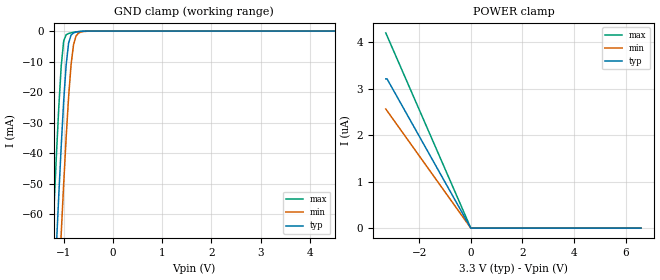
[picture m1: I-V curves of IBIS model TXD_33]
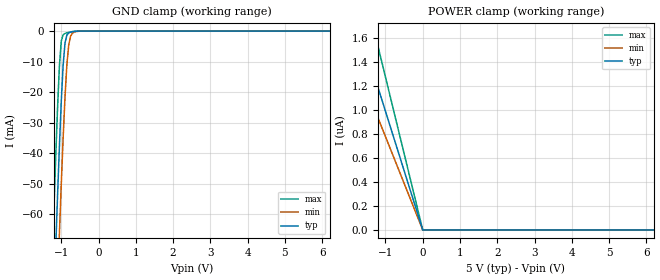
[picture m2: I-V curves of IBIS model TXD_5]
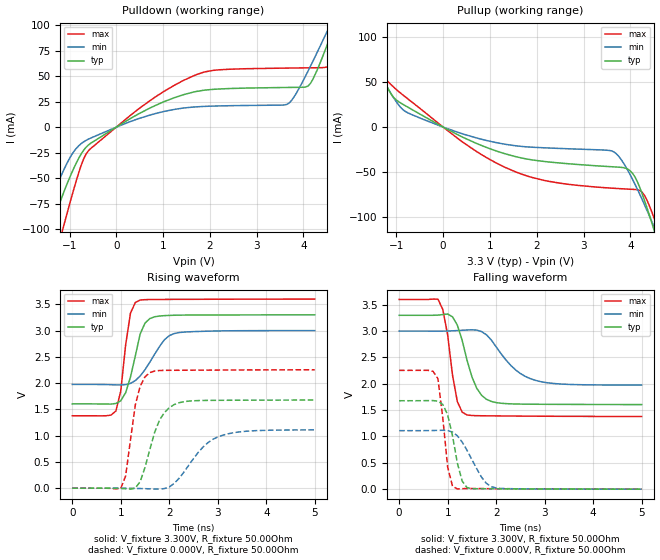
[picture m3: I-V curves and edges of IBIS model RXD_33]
| Texas Instruments Incorporated
| 3000-VRMS Small-Footprint and Low-Power Triple and Quad Channels Digital
| Isolators
| Marketing part#   Digital Voltage Range   Package-type   #pins
| ISO7131CCDBQ   3V - 5.5V   QSOP   16
| ISO7131CCDBQR   3V - 5.5V   QSOP   16
[IBIS Ver]   4.1
[File name]   iso7131.ibs
[File Rev]   1.0
[Date]   04/12/2013
[Source]
| Texas Instruments Incorporated.
| Analog-eLab, HPA
| 12500 TI Blvd
| Dallas, TX -75243
[Notes]   Revision History
| Rev 1.0: 04/12/2013
| - Initial model not matched to silicon
| - C_comp although listed in numberical order of value are
|   obtained from varying PVT conditions.For PVT conditions for
|   eachspecific value, refer to the buffer description under
|   repective [Model].IBIS model user is responsible for using
|   appropriate C_comp to simulate for Signal Integrity.
| - Model names with a trailing _33 contains the model for 3.3V
|   [3.0V and 3.6V]. Model names with a trailing _5 contains the
|   model for 5.0V [4.5V and 5.5V].
[Disclaimer]
| This model is designed as an aid for customers of Texas Instruments.
| TI and its licensors and suppliers make no warranties, either expressed
| or implied, with respect to this  model, including the warranties of
| merchantability or fitness for a particular purpose.
| The model is provided solely on an "as is" basis. The entire risk as to
| its quality and performance is with the customer.
[Copyright] (C)Copyright 2013 Texas Instruments Incorporated.
   All rights reserved.
|   Component ISO7131
[Component]   ISO7131CC
[Manufacturer]  TI
[Package]   |16-pin QSOP  -  DBQ package
|   typ   min   max
R_pkg   0.094432   0.09129   0.09717
L_pkg   1.69628nH   1.65883nH   1.72962nH
C_pkg   0.24832pF   0.2469pF   0.25012pF
[Pin]  signal_name   model_name   R_pin   L_pin   C_pin
1   VCC1   POWER   0.09287  1.67713n  0.24790p
2   GND1   GND   0.05804  1.59222n  0.24871p
3   INA   TXD   0.09129  1.65883n  0.24690p
4   INB   TXD   0.09717  1.72962n  0.24976p
5   OUTC   RXD   0.09664  1.72132n  0.25012p
6   NC   NC   0.03819  1.41587n  0.54383p
7   EN1   NC   0.03819  1.41587n  0.54383p
8   GND1   GND   0.05911  1.64321n  0.24516p
9   GND2   GND   0.05906  1.58357n  0.49660p
10   EN2   NC   0.02805  1.16989n  0.35967p
11   NC   NC   0.02805  1.16989n  0.35967p
12   INC   TXD   0.09546  1.70981n  0.24826p
13   OUTB   RXD   0.09359  1.68659n  0.24766p
14   OUTA   RXD   0.09244  1.67155n  0.24725p
15   GND2   GND   0.03870  1.24255n  0.31586p
16   VCC2   POWER   0.05301  1.30868n  0.31101p
[Model Selector] TXD
TXD_33   TXD Input model for 3.0V - 3.6V
TXD_5   TXD Input model for 4.5V - 5.5V
[Model Selector] RXD
RXD_33   RXD Output model for 3.0V - 3.6V
RXD_5   RXD Output model for 4.5V - 5.5V
| Models and submodels in the file (4): TXD_33 (Input), TXD_5 (Input), RXD_33 (Output), RXD_5 (Output)
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|   TXD_33 Model
[Model]   TXD_33
Model_type   Input
|Signals   TXD
Vinh = 2.0
Vinl = 0.8
|   typ   min   max
|   (nom PVT)   (slow PVT)   (fast PVT)
C_comp   0.6217pF   0.5756pF   0.6712pF
|   typ   min   max
[Voltage Range]   3.3V   3.0V   3.6V
[Temperature Range]   27.0   136.0   -40.0
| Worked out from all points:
|   GND clamp passes 1 mA (typ) near -0.83 V on its own axis
[GND Clamp]
|   Voltage   I(typ)   I(min)   I(max)
-3.3V     -896mA     -941.7mA   -892.3mA
-1.25V    -107.4mA   -137.4mA   -77.4mA
-1.2V     -89.12mA   -119.2mA   -59.18mA
-1.15V    -71.29mA   -101.2mA   -41.62mA
-1.1V     -54.06mA   -83.57mA   -25.26mA
-1.05V    -37.76mA   -66.5mA    -11.46mA
-1V       -23.03mA   -50.19mA   -3.269mA
-950mV    -11.14mA   -35mA      -1.197mA
-900mV    -3.932mA   -21.61mA   -785uA
-800mV    -612.2uA   -4.508mA   -387.7uA
-600mV    -46.68uA   -168.3uA   -47.31uA
6.6V      0A         0A         0A
[POWER Clamp]
|   Voltage   I(typ)   I(min)   I(max)
-3.3V     3.211uA    2.564uA    4.201uA
-3.25V    3.211uA    2.525uA    4.138uA
0V        0A         0A         0A
6.6V      0A         0A         0A
|   TXD_5 Model
[Model]   TXD_5
Model_type   Input
|Signals   TXD
Vinh = 2.0
Vinl = 0.8
|   typ   min   max
|   (nom PVT)   (slow PVT)   (fast PVT)
C_comp   0.5878pF   0.5481pF   0.6309pF
|   typ   min   max
[Voltage Range]   5.0V   4.5V   5.5V
[Temperature Range]   27.0   136.0   -40.0
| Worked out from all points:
|   GND clamp passes 1 mA (typ) near -0.83 V on its own axis
[GND Clamp]
|   Voltage   I(typ)   I(min)   I(max)
-5V       -1.6A      -1.623A    -1.559A
-1.25V    -107.4mA   -137.4mA   -77.4mA
-1.2V     -89.12mA   -119.2mA   -59.18mA
-1.15V    -71.29mA   -101.2mA   -41.62mA
-1.1V     -54.06mA   -83.57mA   -25.26mA
-1.05V    -37.76mA   -66.5mA    -11.46mA
-1V       -23.04mA   -50.19mA   -3.27mA
-950mV    -11.15mA   -35mA      -1.198mA
-850mV    -1.31mA    -11.07mA   -557.5uA
-750mV    -352.2uA   -1.64mA    -261.2uA
-550mV    -20.4uA    -82.68uA   -21.52uA
10V       0A         0A         0A
[POWER Clamp]
|   Voltage   I(typ)   I(min)   I(max)
-5V       4.941uA    3.885uA    6.302uA
-2.15V    2.125uA    1.671uA    2.737uA
-2.1V     2.075uA    1.632uA    2.674uA
-1.7V     1.68uA     1.321uA    2.164uA
-1.65V    1.63uA     1.282uA    2.101uA
-1.3V     1.285uA    1.01uA     1.655uA
0V        0A         0A         0A
10V       0A         0A         0A
|   RXD_33 MODEL
[Model]   RXD_33
Model_type   Output
| Signals   RXD
Vmeas = 1.55V   |Reference voltage for timing measurements
Cref = 15pF   |Timing specification test load capacitance value
| variable   typ   min   max
|   (nom PVT)   (slow PVT)   (fast PVT)
|C_comp Average
C_comp   2.5852pF   2.2483pF   3.0761pF
|C_comp Output Low
|C_comp   2.6504pF   2.3554pF   3.1260pF
|C_comp Output High
|C_comp   2.5200pF   2.1412pF   3.0261pF
|   typ   min   max
[Voltage Range]   3.3V   3.0V   3.6V
[Temperature Range]   27.0   136.0   -40.0
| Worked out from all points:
|   slope of the pulldown table from 0 to 0.495 V, typ, clamps not added: 36.9 ohm
|   slope of the pullup table from 0 to 0.495 V, typ, clamps not added: 38.1 ohm
|   falling waveform, V_fixture 3.300V, R_fixture 50.00Ohm: 20-80 % time 334ps typ, 600ps min, 215ps max; typ from 3.3 V to 1.6 V
|   rising waveform, V_fixture 3.300V, R_fixture 50.00Ohm: 20-80 % time 269ps typ, 440ps min, 178ps max; typ from 1.6 V to 3.3 V
|   rising waveform, V_fixture 0.000V, R_fixture 50.00Ohm: 20-80 % time 354ps typ, 601ps min, 230ps max; typ from 0 V to 1.68 V
|   falling waveform, V_fixture 0.000V, R_fixture 50.00Ohm: 20-80 % time 229ps typ, 400ps min, 158ps max; typ from 1.68 V to 0 V
[Pulldown]
|   Voltage   I(typ)   I(min)   I(max)
-3.3V     -444mA     -323.4mA   -559.5mA
-1.65V    -147.4mA   -102.5mA   -196.8mA
-1.35V    -95.7mA    -66.33mA   -136mA
-1.15V    -67.06mA   -44.62mA   -101.2mA
-600mV    -17.67mA   -11.86mA   -23.39mA
1.65V     34.39mA    19.71mA    50.29mA
3.65V     38.89mA    22.42mA    57.89mA
4.15V     42.92mA    59.74mA    58.14mA
4.55V     85.96mA    98.03mA    60.72mA
4.65V     98.18mA    107.5mA    71.46mA
4.85V     122.5mA    126mA      101.8mA
6.6V      280.4mA    243.7mA    322.1mA
[Pullup]
|   Voltage   I(typ)   I(min)   I(max)
-3.3V     239.5mA    206.9mA    282.1mA
-1.95V    129.9mA    113.6mA    151.3mA
-1.7V     102.1mA    91.19mA    115.7mA
-1.3V     55.75mA    53.78mA    58.94mA
-1V       29.98mA    27.94mA    41.63mA
0V        124.8pA    622.4pA    79.46pA
1.35V     -29.93mA   -19.18mA   -45.19mA
3.65V     -44.04mA   -27.51mA   -67.78mA
4.05V     -51.38mA   -58.2mA    -68.97mA
4.3V      -80.92mA   -85.71mA   -75.5mA
4.55V     -121.4mA   -116mA     -107.4mA
6.6V      -493.8mA   -392mA     -570.7mA
[Ramp]
R_load = 50.00Ohm
|   typ   min   max
dV/dt_r   1.007V/353.701ps 666.318mV/600.696ps   1.353V/229.593ps
dV/dt_f   1.017V/334.234ps 614.806mV/599.733ps   1.333V/215.151ps
[Falling Waveform]
V_fixture = 3.300V
V_fixture_min = 3.000V
V_fixture_max = 3.600V
R_fixture = 50.00Ohm
|   Time   V(typ)   V(min)   V(max)
0s        3.3V       3V         3.6V
800ps     3.304V     3V         3.606V
900ps     3.313V     3V         3.41V
1ns       3.324V     3.001V     2.928V
1.2ns     3.113V     3.01V      1.661V
1.4ns     2.445V     3.021V     1.408V
1.6ns     1.915V     3.019V     1.395V
1.9ns     1.665V     2.831V     1.391V
2.8ns     1.612V     2.068V     1.385V
5ns       1.605V     1.975V     1.379V
[Rising Waveform]
V_fixture = 3.300V
V_fixture_min = 3.000V
V_fixture_max = 3.600V
R_fixture = 50.00Ohm
|   Time   V(typ)   V(min)   V(max)
0s        1.605V     1.975V     1.379V
900ps     1.613V     1.967V     1.471V
1ns       1.664V     1.965V     1.851V
1.1ns     1.817V     1.971V     2.723V
1.2ns     2.114V     1.995V     3.333V
1.4ns     2.937V     2.136V     3.582V
1.6ns     3.229V     2.4V       3.591V
1.9ns     3.284V     2.825V     3.593V
2.1ns     3.292V     2.943V     3.594V
5ns       3.3V       3V         3.6V
[Rising Waveform]
V_fixture = 0.000V
V_fixture_min = 0.000V
V_fixture_max = 0.000V
R_fixture = 50.00Ohm
|   Time   V(typ)   V(min)   V(max)
0s        336.7pV    705.2pV    374.2pV
1ns       -5.097mV   157.2uV    -2.804mV
1.1ns     -10.77mV   -533.8uV   231mV
1.3ns     2.172mV    -3.954mV   1.586V
1.4ns     125.6mV    -6.338mV   1.939V
1.6ns     740.1mV    -11.61mV   2.201V
1.8ns     1.298V     -16.07mV   2.24V
2.2ns     1.626V     186mV      2.245V
3ns       1.673V     975.1mV    2.249V
5ns       1.678V     1.111V     2.254V
[Falling Waveform]
V_fixture = 0.000V
V_fixture_min = 0.000V
V_fixture_max = 0.000V
R_fixture = 50.00Ohm
|   Time   V(typ)   V(min)   V(max)
0s        1.678V     1.111V     2.254V
700ps     1.681V     1.113V     2.235V
800ps     1.67V      1.116V     2.097V
1ns       1.412V     1.112V     422.2mV
1.1ns     1.014V     1.084V     56.58mV
1.2ns     495.5mV    1.013V     4.556mV
1.3ns     153.7mV    894mV      9.242mV
1.4ns     30.49mV    736.9mV    12.55mV
1.9ns     7.265mV    47.26mV    9.425mV
5ns       336.7pV    705.2pV    374.2pV
